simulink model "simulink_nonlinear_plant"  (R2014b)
settings: Solver=ode45  StartTime=0.0  StopTime=10.0  RelTol=1e-3

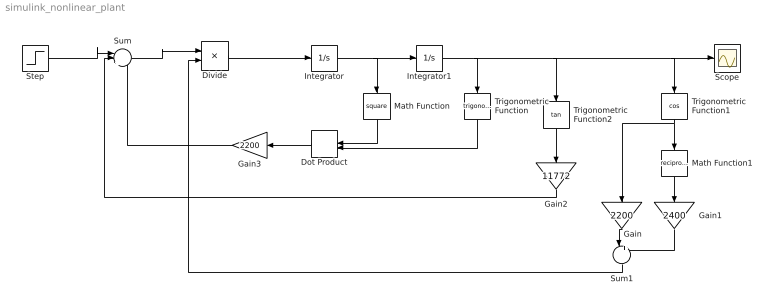
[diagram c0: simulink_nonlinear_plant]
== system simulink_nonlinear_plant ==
  Divide : Product  Inputs=*/
  Dot Product : DotProduct
  Gain : Gain  Gain=2200
  Gain1 : Gain  Gain=2400
  Gain2 : Gain  Gain=11772
  Gain3 : Gain  Gain=2200
  Integrator : Integrator
  Integrator1 : Integrator
  Math Function : Math  Operator=square
  Math Function1 : Math  Operator=reciprocal
  Scope : Scope
  Step : Step  SampleTime=0
  Sum : Sum  Inputs=|+++
  Sum1 : Sum  Inputs=|+-
  Trigonometric Function : Trigonometry
  Trigonometric Function1 : Trigonometry  Operator=cos
  Trigonometric Function2 : Trigonometry  Operator=tan
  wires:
  Step/1 -> Sum/1
  Sum/1 -> Divide/1
  Divide/1 -> Integrator/1
  Integrator/1 -> Math Function/1, Integrator1/1
  Integrator1/1 -> Scope/1, Trigonometric Function1/1, Trigonometric Function2/1, Trigonometric Function/1
  Math Function/1 -> Dot Product/1
  Trigonometric Function/1 -> Dot Product/2
  Dot Product/1 -> Gain3/1
  Trigonometric Function1/1 -> Gain/1, Math Function1/1
  Math Function1/1 -> Gain1/1
  Gain/1 -> Sum1/1
  Gain1/1 -> Sum1/2
  Sum1/1 -> Divide/2
  Trigonometric Function2/1 -> Gain2/1
  Gain2/1 -> Sum/2
  Gain3/1 -> Sum/3
